| IBIS file stm32u595_599_5a5_5a9_tfbga169.ibs
[IBIS ver] 4.2
[File name] stm32u595_599_5a5_5a9_tfbga169.ibs
[File Rev] rev2.0
[Date]  11-09-2023
[Source] Data Created at STMicroelectronics
[Notes]  File originated from ELDO simulations.
[Disclaimer]  This information is for modeling purpose only and is
   not guaranteed. The information is subject to change without
   notice.
[Copyright] Copyright 2023 STMicroelectronics Inc.
|   Component stm32u595_599_5a5_5a9_tfbga169
[Component] stm32u595_599_5a5_5a9_tfbga169
[Manufacturer] STMicroelectronics
[Package]
| variable   typ   min   max
R_pkg  0  NA  NA
L_pkg  0  NA  NA
C_pkg  0  NA  NA
[Pin]   signal_name   model_name
A1  PE2  io8_100m_hslv_ft
A2  PI6  io8_spi_ft
A3  VDD  power
A4  VCAP  nc
A5  PG15  io8_100m_hslv_ft
A6  VDDIO2  power
A7  PG9  io8_100m_hslv_ft
A8  VDD  power
A9  PC11  io8_100m_hslv_ft
A10  PA15  nc
A11  VDD  power
A12  PI1  io8_spi_ft
A13  PH15  io8_spi_ft
B1  VDD  power
B2  VSS  gnd
B3  PI5  io8_100m_hslv_ft
B4  VSS  gnd
B5  PB6  io8_100m_i2c_ft
B6  PB4  io8_100m_i2c_ft
B7  PD6  io8_166m_hslv_ft
B8  VSS  gnd
B9  PD0  io8_100m_hslv_ft
B10  PI4  io8_spi_ft
B11  VSS  gnd
B12  PI0  io8_spi_ft
B13  PH12  io8_spi_ft
C1  VBAT  power
C2  PE4  io8_100m_hslv_tamp_ft
C3  PI7  io8_spi_ft
C4  PE1  io8_100m_hslv_ft
C5  PH3-BOOT0  nc
C6  PB5  io8_166m_hslv_ft
C7  PG10  io8_100m_hslv_ft
C8  PD4  io8_100m_hslv_ft
C9  PC10  io8_100m_ft
C10  PA14  io8_100m_ft
C11  PH14  io8_spi_ft
C12  PH13  io8_spi_ft
C13  PH10  io8_spi_ft
D1  PC14-OSC32_IN   nc
D2  PE5  io8_100m_hslv_tamp_ft
D3  PE3  io8_100m_hslv_tamp_ft
D4  PE0  io8_100m_hslv_ft
D5  PB9  io8_100m_i2c_ft
D6  PB3  io8_100m_i2c_ft
D7  PD7  io8_100m_hslv_ft
D8  PD3  io8_166m_hslv_ft
D9  PH11  io8_spi_ft
D10  PI3  io8_spi_ft
D11  PI2  io8_spi_ft
D12  PH8  io8_100m_hslv_ft
D13  VDD  power
E1  PC15-OSC32_OUT   nc
E2  PF0  io8_100m_hslv_ft
E3  PC13  io8_100m_ft
E4  PE6  io8_100m_hslv_tamp_ft
E5  PB8  io8_100m_i2c_ft
E6  PG12  io8_100m_hslv_ft
E7  PD5  io8_100m_hslv_ft
E8  PC12  io8_166m_hslv_ft
E9  PH9  io8_spi_ft
E10  PH4  io8_100m_hslv_ft
E11  PH6  io8_166m_hslv_ft
E12  VSS  gnd
E13  VDDUSB  power
F1  PF8  io8_100m_hslv_ft
F2  VSS  gnd
F3  PF1  io8_100m_hslv_ft
F4  PF2  io8_100m_hslv_ft
F5  PB7  io8_spi_hslv_ft
F6  PD1  io8_100m_hslv_ft
F7  PD2  io8_100m_ft
F8  PH7  io8_spi_hslv_ft
F9  PH5  io8_100m_i2c_ft
F10  PH2  io8_100m_hslv_ft
F11  PA10  io8_100m_usb_id
F12  PA13  io8_100m_ft
F13  PA12  io8_100m_ft
G1  VDD  power
G2  PF7  io8_100m_hslv_ft
G3  PF9  io8_100m_hslv_ft
G4  PF5  io8_spi_ft
G5  PF3  io8_100m_hslv_ft
G6  PF4  io8_spi_ft
G7  PA8  io8_166m_hslv_ft
G8  PG7  io8_100m_hslv_ft
G9  PC9  io8_100m_ft
G10  PC8  io8_100m_ft
G11  PA9  io8_100m_usb_vbus_ft
G12  PC7  io8_100m_ft
G13  PA11  io8_100m_ft
H1  PH0-OSC_IN  nc
H2  VSS  gnd
H3  NRST  nc
H4  PF10  io8_166m_hslv_ft
H5  OPAMP2_VINM  nc
H6  PF6  io8_100m_hslv_ft
H7  PG1  io8_100m_hslv_ft
H8  PE10  io8_166m_hslv_ft
H9  PG8  io8_100m_i2c_ft
H10  PG6  io8_100m_hslv_ft
H11  PG4  io8_100m_hslv_ft
H12  VDDIO2  power
H13  PC6  io8_100m_ft
J1  PH1-OSC_OUT   nc
J2  PC0  io8_100m_hslv_ft
J3  PC1  io8_spi_hslv_ft
J4  PC2  io8_100m_hslv_ft
J5  PA7  io8_100m_hslv_ft
J6  PG0  io8_100m_hslv_ft
J7  PE9  io8_166m_hslv_ft
J8  PG3  io8_100m_hslv_ft
J9  PG5  io8_100m_hslv_ft
J10  PD14  io8_100m_hslv_ft
J11  PD15  io8_100m_hslv_ft
J12  VSS  gnd
J13  VDD  power
K1  PC3  io8_100m_hslv_ft
K2  VSSA  nc
K3  PA0  io8_100m_hslv_tamp_ft
K4  PA5  io8_100m_ft
K5  PB0  io8_100m_hslv_ft
K6  PF12  io8_100m_hslv_ft
K7  PE8  io8_100m_hslv_ft
K8  PE14  io8_100m_hslv_ft
K9  PB10  io8_spi_hslv_ft
K10  PD12  io8_100m_hslv_ft
K11  PD10  io8_100m_hslv_ft
K12  PD13  io8_100m_hslv_ft
K13  PG2  io8_100m_hslv_ft
L1  VREFP  nc
L2  VDDA  nc
L3  PA1  io8_100m_hslv_tamp_ft
L4  PC4  io8_100m_hslv_ft
L5  PB2  io8_100m_hslv_tamp_ft
L6  PF14  io8_100m_hslv_ft
L7  PE7  io8_100m_hslv_ft
L8  PE13  io8_100m_hslv_ft
L9  PB11  io8_100m_hslv_ft
L10  PB12  io8_166m_hslv_ft
L11  PB15  nc
L12  PD8  io8_100m_hslv_ft
L13  PD9  io8_100m_hslv_ft
M1  OPAMP1_VINM  nc
M2  PA2  io8_100m_hslv_ft
M3  VSS  gnd
M4  PC5  io8_100m_tamp_ft
M5  PF11  io8_166m_hslv_ft
M6  PF13  io8_100m_hslv_ft
M7  VSS  gnd
M8  PE11  io8_100m_hslv_ft
M9  PE15  io8_100m_hslv_ft
M10  PG11  io8_100m_hslv_ft
M11  VSS  gnd
M12  PB14  io8_100m_i2c_ft
M13  PD11  io8_100m_hslv_ft
N1  PA4  io8_100m_hslv_ft
N2  PA3  io8_166m_hslv_ft
N3  VDD  power
N4  PA6  io8_100m_hslv_ft
N5  PB1  io8_100m_hslv_ft
N6  PF15  io8_100m_hslv_ft
N7  VDD  power
N8  PE12  io8_100m_hslv_ft
N9  PG14  io8_100m_hslv_ft
N10  PG13  io8_100m_hslv_ft
N11  VCAP  nc
N12  VDD  power
N13  PB13  io8_100m_i2c_ft
[Package Model]   481-tfbga-7x7-ldo-169-220908
[Pin Mapping]   pulldown_ref   pullup_ref   | Comment
A1  gndio  vddiom
A2  gndio  vddiom
A3  nc  vddiom
A4  nc  nc
A5  gndio  vddiom  | Depending on IO usage
| A5  gndio  vddio2  | Depending on IO usage
A6  nc  vddio2
A7  gndio  vddiom  | Depending on IO usage
| A7  gndio  vddio2  | Depending on IO usage
A8  nc  vddiom
A9  gndio  vddiom
A10  nc  nc
A11  nc  vddiom
A12  gndio  vddiom
A13  gndio  vddiom
B1  nc  vddiom
B2  gndio  nc
B3  gndio  vddiom
B4  gndio  nc
B5  gndio  vddiom
B6  gndio  vddiom
B7  gndio  vddiom
B8  gndio  nc
B9  gndio  vddiom
B10  gndio  vddiom
B11  gndio  nc
B12  gndio  vddiom
B13  gndio  vddiom
C1  nc  vsw
C2  gndio  vddiom
C3  gndio  vddiom
C4  gndio  vddiom
C5  nc  nc
C6  gndio  vddiom
C7  gndio  vddiom  | Depending on IO usage
| C7  gndio  vddio2  | Depending on IO usage
C8  gndio  vddiom
C9  gndio  vddiom
C10  gndio  vddiom
C11  gndio  vddiom
C12  gndio  vddiom
C13  gndio  vddiom
D1  nc  nc
D2  gndio  vddiom
D3  gndio  vddiom
D4  gndio  vddiom
D5  gndio  vddiom
D6  gndio  vddiom
D7  gndio  vddiom
D8  gndio  vddiom
D9  gndio  vddiom
D10  gndio  vddiom
D11  gndio  vddiom
D12  gndio  vddiom
D13  nc  vddiom
E1  nc  nc
E2  gndio  vddiom
E3  gndio  vddiom  | Depending on IO usage
| E3  gndio  vsw  | Depending on IO usage
E4  gndio  vddiom
E5  gndio  vddiom
E6  gndio  vddiom  | Depending on IO usage
| E6  gndio  vddio2  | Depending on IO usage
E7  gndio  vddiom
E8  gndio  vddiom
E9  gndio  vddiom
E10  gndio  vddiom
E11  gndio  vddiom
E12  gndio  nc
E13  nc  vddusb
F1  gndio  vddiom
F2  gndio  nc
F3  gndio  vddiom
F4  gndio  vddiom
F5  gndio  vddiom
F6  gndio  vddiom
F7  gndio  vddiom
F8  gndio  vddiom
F9  gndio  vddiom
F10  gndio  vddiom
F11  gndio  vddiom  | Depending on IO usage
| F11  gndio  vddusb  | Depending on IO usage
F12  gndio  vddiom  | Depending on IO usage
| F12  gndio  vddusb  | Depending on IO usage
F13  gndio  vddiom  | Depending on IO usage
| F13  gndio  vddusb  | Depending on IO usage
G1  nc  vddiom
G2  gndio  vddiom
G3  gndio  vddiom
G4  gndio  vddiom
G5  gndio  vddiom
G6  gndio  vddiom
G7  gndio  vddiom
G8  gndio  vddiom  | Depending on IO usage
| G8  gndio  vddio2  | Depending on IO usage
G9  gndio  vddiom
G10  gndio  vddiom
G11  gndio  vddiom  | Depending on IO usage
| G11  gndio  vddusb  | Depending on IO usage
G12  gndio  vddiom
G13  gndio  vddiom  | Depending on IO usage
| G13  gndio  vddusb  | Depending on IO usage
H1  nc  nc
H2  gndio  nc
H3  nc  nc
H4  gndio  vddiom
H5  nc  nc
H6  gndio  vddiom
H7  gndio  vddiom
H8  gndio  vddiom
H9  gndio  vddiom  | Depending on IO usage
| H9  gndio  vddio2  | Depending on IO usage
H10  gndio  vddiom  | Depending on IO usage
| H10  gndio  vddio2  | Depending on IO usage
H11  gndio  vddiom  | Depending on IO usage
| H11  gndio  vddio2  | Depending on IO usage
H12  nc  vddio2
H13  gndio  vddiom
J1  nc  nc
J2  gndio  vddiom
J3  gndio  vddiom
J4  gndio  vddiom
J5  gndio  vddiom
J6  gndio  vddiom
J7  gndio  vddiom
J8  gndio  vddiom  | Depending on IO usage
| J8  gndio  vddio2  | Depending on IO usage
J9  gndio  vddiom  | Depending on IO usage
| J9  gndio  vddio2  | Depending on IO usage
J10  gndio  vddiom
J11  gndio  vddiom
J12  gndio  nc
J13  nc  vddiom
K1  gndio  vddiom
K2  nc  nc
K3  gndio  vddiom
K4  gndio  vddiom
K5  gndio  vddiom
K6  gndio  vddiom
K7  gndio  vddiom
K8  gndio  vddiom
K9  gndio  vddiom
K10  gndio  vddiom
K11  gndio  vddiom
K12  gndio  vddiom
K13  gndio  vddiom  | Depending on IO usage
| K13  gndio  vddio2  | Depending on IO usage
L1  nc  nc
L2  nc  nc
L3  gndio  vddiom
L4  gndio  vddiom
L5  gndio  vddiom
L6  gndio  vddiom
L7  gndio  vddiom
L8  gndio  vddiom
L9  gndio  vddiom
L10  gndio  vddiom
L11  nc  nc
L12  gndio  vddiom
L13  gndio  vddiom
M1  nc  nc
M2  gndio  vddiom
M3  gndio  nc
M4  gndio  vddiom
M5  gndio  vddiom
M6  gndio  vddiom
M7  gndio  nc
M8  gndio  vddiom
M9  gndio  vddiom
M10  gndio  vddiom  | Depending on IO usage
| M10  gndio  vddio2  | Depending on IO usage
M11  gndio  nc
M12  gndio  vddiom
M13  gndio  vddiom
N1  gndio  vddiom
N2  gndio  vddiom
N3  nc  vddiom
N4  gndio  vddiom
N5  gndio  vddiom
N6  gndio  vddiom
N7  nc  vddiom
N8  gndio  vddiom
N9  gndio  vddiom  | Depending on IO usage
| N9  gndio  vddio2  | Depending on IO usage
N10  gndio  vddiom  | Depending on IO usage
| N10  gndio  vddio2  | Depending on IO usage
N11  nc  nc
N12  nc  vddiom
N13  gndio  vddiom
[Model Selector] io8_100m_ft
io8_100m_ft_hs_1v2  "IO8_FT 100MHz high speed @ 1.2V"
io8_100m_ft_fs_1v2  "IO8_FT 100MHz fast speed @ 1.2V"
io8_100m_ft_fs_pd_1v2  "IO8_FT 100MHz fast speed @ 1.2V pulldown"
io8_100m_ft_ms_1v2  "IO8_FT 100MHz med speed @ 1.2V"
io8_100m_ft_ms_pd_1v2  "IO8_FT 100MHz med speed @ 1.2V pulldown"
io8_100m_ft_ls_1v2  "IO8_FT 100MHz low speed @ 1.2V"
io8_100m_ft_ls_pd_1v2  "IO8_FT 100MHz low speed @ 1.2V pulldown"
io8_100m_ft_hs_1v8  "IO8_FT 100MHz high speed @ 1.8V"
io8_100m_ft_hs_pd_1v8  "IO8_FT 100MHz high speed @ 1.8V pulldown"
io8_100m_ft_fs_1v8  "IO8_FT 100MHz fast speed @ 1.8V"
io8_100m_ft_fs_pd_1v8  "IO8_FT 100MHz fast speed @ 1.8V pulldown"
io8_100m_ft_ms_1v8  "IO8_FT 100MHz med speed @ 1.8V"
io8_100m_ft_ms_pd_1v8  "IO8_FT 100MHz med speed @ 1.8V pulldown"
io8_100m_ft_ls_1v8  "IO8_FT 100MHz low speed @ 1.8V"
io8_100m_ft_ls_pd_1v8  "IO8_FT 100MHz low speed @ 1.8V pulldown"
io8_100m_ft_hs_3v3  "IO8_FT 100MHz high speed @ 3.3V"
io8_100m_ft_hs_pd_3v3  "IO8_FT 100MHz high speed @ 3.3V pulldown"
io8_100m_ft_fs_3v3  "IO8_FT 100MHz fast speed @ 3.3V"
io8_100m_ft_fs_pd_3v3  "IO8_FT 100MHz fast speed @ 3.3V pulldown"
io8_100m_ft_ms_3v3  "IO8_FT 100MHz med speed @ 3.3V"
io8_100m_ft_ms_pd_3v3  "IO8_FT 100MHz med speed @ 3.3V pulldown"
io8_100m_ft_ls_3v3  "IO8_FT 100MHz low speed @ 3.3V"
io8_100m_ft_ls_pd_3v3  "IO8_FT 100MHz low speed @ 3.3V pulldown"
[Model Selector] io8_100m_hslv_ft
io8_100m_ft_hs_1v2  "IO8_FT 100MHz high speed @ 1.2V"
io8_100m_ft_hs_pu_1v2  "IO8_FT 100MHz high speed @ 1.2V pullup"
io8_100m_ft_hs_pd_1v2  "IO8_FT 100MHz high speed @ 1.2V pulldown"
io8_100m_ft_fs_1v2  "IO8_FT 100MHz fast speed @ 1.2V"
io8_100m_ft_fs_pu_1v2  "IO8_FT 100MHz fast speed @ 1.2V pullup"
io8_100m_ft_fs_pd_1v2  "IO8_FT 100MHz fast speed @ 1.2V pulldown"
io8_100m_ft_ms_1v2  "IO8_FT 100MHz med speed @ 1.2V"
io8_100m_ft_ms_pu_1v2  "IO8_FT 100MHz med speed @ 1.2V pullup"
io8_100m_ft_ms_pd_1v2  "IO8_FT 100MHz med speed @ 1.2V pulldown"
io8_100m_ft_ls_1v2  "IO8_FT 100MHz low speed @ 1.2V"
io8_100m_ft_ls_pu_1v2  "IO8_FT 100MHz low speed @ 1.2V pullup"
io8_100m_ft_ls_pd_1v2  "IO8_FT 100MHz low speed @ 1.2V pulldown"
io8_100m_ft_hs_1v8  "IO8_FT 100MHz high speed @ 1.8V"
io8_100m_ft_hs_pu_1v8  "IO8_FT 100MHz high speed @ 1.8V pullup"
io8_100m_ft_hs_pd_1v8  "IO8_FT 100MHz high speed @ 1.8V pulldown"
io8_100m_ft_fs_1v8  "IO8_FT 100MHz fast speed @ 1.8V"
io8_100m_ft_fs_pu_1v8  "IO8_FT 100MHz fast speed @ 1.8V pullup"
io8_100m_ft_fs_pd_1v8  "IO8_FT 100MHz fast speed @ 1.8V pulldown"
io8_100m_ft_ms_1v8  "IO8_FT 100MHz med speed @ 1.8V"
io8_100m_ft_ms_pu_1v8  "IO8_FT 100MHz med speed @ 1.8V pullup"
io8_100m_ft_ms_pd_1v8  "IO8_FT 100MHz med speed @ 1.8V pulldown"
io8_100m_ft_ls_1v8  "IO8_FT 100MHz low speed @ 1.8V"
io8_100m_ft_ls_pu_1v8  "IO8_FT 100MHz low speed @ 1.8V pullup"
io8_100m_ft_ls_pd_1v8  "IO8_FT 100MHz low speed @ 1.8V pulldown"
io8_100m_ft_hs_3v3  "IO8_FT 100MHz high speed @ 3.3V"
io8_100m_ft_hs_pu_3v3  "IO8_FT 100MHz high speed @ 3.3V pullup"
io8_100m_ft_hs_pd_3v3  "IO8_FT 100MHz high speed @ 3.3V pulldown"
io8_100m_ft_fs_3v3  "IO8_FT 100MHz fast speed @ 3.3V"
io8_100m_ft_fs_pu_3v3  "IO8_FT 100MHz fast speed @ 3.3V pullup"
io8_100m_ft_fs_pd_3v3  "IO8_FT 100MHz fast speed @ 3.3V pulldown"
io8_100m_ft_ms_3v3  "IO8_FT 100MHz med speed @ 3.3V"
io8_100m_ft_ms_pu_3v3  "IO8_FT 100MHz med speed @ 3.3V pullup"
io8_100m_ft_ms_pd_3v3  "IO8_FT 100MHz med speed @ 3.3V pulldown"
io8_100m_ft_ls_3v3  "IO8_FT 100MHz low speed @ 3.3V"
io8_100m_ft_ls_pu_3v3  "IO8_FT 100MHz low speed @ 3.3V pullup"
io8_100m_ft_ls_pd_3v3  "IO8_FT 100MHz low speed @ 3.3V pulldown"
io8_100m_hslv_ft_hs_1v2  "IO8_FT 100MHz HSLV high speed @ 1.2V"
io8_100m_hslv_ft_hs_pu_1v2  "IO8_FT 100MHz HSLV high speed @ 1.2V pullup"
io8_100m_hslv_ft_hs_pd_1v2  "IO8_FT 100MHz HSLV high speed @ 1.2V pulldown"
io8_100m_hslv_ft_fs_1v2  "IO8_FT 100MHz HSLV fast speed @ 1.2V"
io8_100m_hslv_ft_fs_pu_1v2  "IO8_FT 100MHz HSLV fast speed @ 1.2V pullup"
io8_100m_hslv_ft_fs_pd_1v2  "IO8_FT 100MHz HSLV fast speed @ 1.2V pulldown"
io8_100m_hslv_ft_ms_1v2  "IO8_FT 100MHz HSLV med speed @ 1.2V"
io8_100m_hslv_ft_ms_pu_1v2  "IO8_FT 100MHz HSLV med speed @ 1.2V pullup"
io8_100m_hslv_ft_ms_pd_1v2  "IO8_FT 100MHz HSLV med speed @ 1.2V pulldown"
io8_100m_hslv_ft_ls_1v2  "IO8_FT 100MHz HSLV low speed @ 1.2V"
io8_100m_hslv_ft_ls_pu_1v2  "IO8_FT 100MHz HSLV low speed @ 1.2V pullup"
io8_100m_hslv_ft_ls_pd_1v2  "IO8_FT 100MHz HSLV low speed @ 1.2V pulldown"
io8_100m_hslv_ft_hs_1v8  "IO8_FT 100MHz HSLV high speed @ 1.8V"
io8_100m_hslv_ft_hs_pu_1v8  "IO8_FT 100MHz HSLV high speed @ 1.8V pullup"
io8_100m_hslv_ft_hs_pd_1v8  "IO8_FT 100MHz HSLV high speed @ 1.8V pulldown"
io8_100m_hslv_ft_fs_1v8  "IO8_FT 100MHz HSLV fast speed @ 1.8V"
io8_100m_hslv_ft_fs_pu_1v8  "IO8_FT 100MHz HSLV fast speed @ 1.8V pullup"
io8_100m_hslv_ft_fs_pd_1v8  "IO8_FT 100MHz HSLV fast speed @ 1.8V pulldown"
io8_100m_hslv_ft_ms_1v8  "IO8_FT 100MHz HSLV med speed @ 1.8V"
io8_100m_hslv_ft_ms_pu_1v8  "IO8_FT 100MHz HSLV med speed @ 1.8V pullup"
io8_100m_hslv_ft_ms_pd_1v8  "IO8_FT 100MHz HSLV med speed @ 1.8V pulldown"
io8_100m_hslv_ft_ls_1v8  "IO8_FT 100MHz HSLV low speed @ 1.8V"
io8_100m_hslv_ft_ls_pu_1v8  "IO8_FT 100MHz HSLV low speed @ 1.8V pullup"
io8_100m_hslv_ft_ls_pd_1v8  "IO8_FT 100MHz HSLV low speed @ 1.8V pulldown"
io8_100m_hslv_ft_hs_2v5  "IO8_FT 100MHz HSLV high speed @ 2.5V"
io8_100m_hslv_ft_hs_pu_2v5  "IO8_FT 100MHz HSLV high speed @ 2.5V pullup"
io8_100m_hslv_ft_hs_pd_2v5  "IO8_FT 100MHz HSLV high speed @ 2.5V pulldown"
io8_100m_hslv_ft_fs_2v5  "IO8_FT 100MHz HSLV fast speed @ 2.5V"
io8_100m_hslv_ft_fs_pu_2v5  "IO8_FT 100MHz HSLV fast speed @ 2.5V pullup"
io8_100m_hslv_ft_fs_pd_2v5  "IO8_FT 100MHz HSLV fast speed @ 2.5V pulldown"
io8_100m_hslv_ft_ms_2v5  "IO8_FT 100MHz HSLV med speed @ 2.5V"
io8_100m_hslv_ft_ms_pu_2v5  "IO8_FT 100MHz HSLV med speed @ 2.5V pullup"
io8_100m_hslv_ft_ms_pd_2v5  "IO8_FT 100MHz HSLV med speed @ 2.5V pulldown"
io8_100m_hslv_ft_ls_2v5  "IO8_FT 100MHz HSLV low speed @ 2.5V"
io8_100m_hslv_ft_ls_pu_2v5  "IO8_FT 100MHz HSLV low speed @ 2.5V pullup"
io8_100m_hslv_ft_ls_pd_2v5  "IO8_FT 100MHz HSLV low speed @ 2.5V pulldown"
[Model Selector] io8_100m_hslv_tamp_ft
io8_100m_ft_hs_1v2  "IO8_FT 100MHz high speed @ 1.2V"
io8_100m_ft_hs_pu_1v2  "IO8_FT 100MHz high speed @ 1.2V pullup"
io8_100m_ft_hs_pd_1v2  "IO8_FT 100MHz high speed @ 1.2V pulldown"
io8_100m_ft_fs_1v2  "IO8_FT 100MHz fast speed @ 1.2V"
io8_100m_ft_fs_pu_1v2  "IO8_FT 100MHz fast speed @ 1.2V pullup"
io8_100m_ft_fs_pd_1v2  "IO8_FT 100MHz fast speed @ 1.2V pulldown"
io8_100m_ft_ms_1v2  "IO8_FT 100MHz med speed @ 1.2V"
io8_100m_ft_ms_pu_1v2  "IO8_FT 100MHz med speed @ 1.2V pullup"
io8_100m_ft_ms_pd_1v2  "IO8_FT 100MHz med speed @ 1.2V pulldown"
io8_100m_ft_ls_1v2  "IO8_FT 100MHz low speed @ 1.2V"
io8_100m_ft_ls_pu_1v2  "IO8_FT 100MHz low speed @ 1.2V pullup"
io8_100m_ft_ls_pd_1v2  "IO8_FT 100MHz low speed @ 1.2V pulldown"
io8_100m_ft_hs_1v8  "IO8_FT 100MHz high speed @ 1.8V"
io8_100m_ft_hs_pu_1v8  "IO8_FT 100MHz high speed @ 1.8V pullup"
io8_100m_ft_hs_pd_1v8  "IO8_FT 100MHz high speed @ 1.8V pulldown"
io8_100m_ft_fs_1v8  "IO8_FT 100MHz fast speed @ 1.8V"
io8_100m_ft_fs_pu_1v8  "IO8_FT 100MHz fast speed @ 1.8V pullup"
io8_100m_ft_fs_pd_1v8  "IO8_FT 100MHz fast speed @ 1.8V pulldown"
io8_100m_ft_ms_1v8  "IO8_FT 100MHz med speed @ 1.8V"
io8_100m_ft_ms_pu_1v8  "IO8_FT 100MHz med speed @ 1.8V pullup"
io8_100m_ft_ms_pd_1v8  "IO8_FT 100MHz med speed @ 1.8V pulldown"
io8_100m_ft_ls_1v8  "IO8_FT 100MHz low speed @ 1.8V"
io8_100m_ft_ls_pu_1v8  "IO8_FT 100MHz low speed @ 1.8V pullup"
io8_100m_ft_ls_pd_1v8  "IO8_FT 100MHz low speed @ 1.8V pulldown"
io8_100m_ft_hs_3v3  "IO8_FT 100MHz high speed @ 3.3V"
io8_100m_ft_hs_pu_3v3  "IO8_FT 100MHz high speed @ 3.3V pullup"
io8_100m_ft_hs_pd_3v3  "IO8_FT 100MHz high speed @ 3.3V pulldown"
io8_100m_ft_fs_3v3  "IO8_FT 100MHz fast speed @ 3.3V"
io8_100m_ft_fs_pu_3v3  "IO8_FT 100MHz fast speed @ 3.3V pullup"
io8_100m_ft_fs_pd_3v3  "IO8_FT 100MHz fast speed @ 3.3V pulldown"
io8_100m_ft_ms_3v3  "IO8_FT 100MHz med speed @ 3.3V"
io8_100m_ft_ms_pu_3v3  "IO8_FT 100MHz med speed @ 3.3V pullup"
io8_100m_ft_ms_pd_3v3  "IO8_FT 100MHz med speed @ 3.3V pulldown"
io8_100m_ft_ls_3v3  "IO8_FT 100MHz low speed @ 3.3V"
io8_100m_ft_ls_pu_3v3  "IO8_FT 100MHz low speed @ 3.3V pullup"
io8_100m_ft_ls_pd_3v3  "IO8_FT 100MHz low speed @ 3.3V pulldown"
io8_100m_hslv_ft_hs_1v2  "IO8_FT 100MHz HSLV high speed @ 1.2V"
io8_100m_hslv_ft_hs_pu_1v2  "IO8_FT 100MHz HSLV high speed @ 1.2V pullup"
io8_100m_hslv_ft_hs_pd_1v2  "IO8_FT 100MHz HSLV high speed @ 1.2V pulldown"
io8_100m_hslv_ft_fs_1v2  "IO8_FT 100MHz HSLV fast speed @ 1.2V"
io8_100m_hslv_ft_fs_pu_1v2  "IO8_FT 100MHz HSLV fast speed @ 1.2V pullup"
io8_100m_hslv_ft_fs_pd_1v2  "IO8_FT 100MHz HSLV fast speed @ 1.2V pulldown"
io8_100m_hslv_ft_ms_1v2  "IO8_FT 100MHz HSLV med speed @ 1.2V"
io8_100m_hslv_ft_ms_pu_1v2  "IO8_FT 100MHz HSLV med speed @ 1.2V pullup"
io8_100m_hslv_ft_ms_pd_1v2  "IO8_FT 100MHz HSLV med speed @ 1.2V pulldown"
io8_100m_hslv_ft_ls_1v2  "IO8_FT 100MHz HSLV low speed @ 1.2V"
io8_100m_hslv_ft_ls_pu_1v2  "IO8_FT 100MHz HSLV low speed @ 1.2V pullup"
io8_100m_hslv_ft_ls_pd_1v2  "IO8_FT 100MHz HSLV low speed @ 1.2V pulldown"
io8_100m_hslv_ft_hs_1v8  "IO8_FT 100MHz HSLV high speed @ 1.8V"
io8_100m_hslv_ft_hs_pu_1v8  "IO8_FT 100MHz HSLV high speed @ 1.8V pullup"
io8_100m_hslv_ft_hs_pd_1v8  "IO8_FT 100MHz HSLV high speed @ 1.8V pulldown"
io8_100m_hslv_ft_fs_1v8  "IO8_FT 100MHz HSLV fast speed @ 1.8V"
io8_100m_hslv_ft_fs_pu_1v8  "IO8_FT 100MHz HSLV fast speed @ 1.8V pullup"
io8_100m_hslv_ft_fs_pd_1v8  "IO8_FT 100MHz HSLV fast speed @ 1.8V pulldown"
io8_100m_hslv_ft_ms_1v8  "IO8_FT 100MHz HSLV med speed @ 1.8V"
io8_100m_hslv_ft_ms_pu_1v8  "IO8_FT 100MHz HSLV med speed @ 1.8V pullup"
io8_100m_hslv_ft_ms_pd_1v8  "IO8_FT 100MHz HSLV med speed @ 1.8V pulldown"
io8_100m_hslv_ft_ls_1v8  "IO8_FT 100MHz HSLV low speed @ 1.8V"
io8_100m_hslv_ft_ls_pu_1v8  "IO8_FT 100MHz HSLV low speed @ 1.8V pullup"
io8_100m_hslv_ft_ls_pd_1v8  "IO8_FT 100MHz HSLV low speed @ 1.8V pulldown"
io8_100m_hslv_ft_hs_2v5  "IO8_FT 100MHz HSLV high speed @ 2.5V"
io8_100m_hslv_ft_hs_pu_2v5  "IO8_FT 100MHz HSLV high speed @ 2.5V pullup"
io8_100m_hslv_ft_hs_pd_2v5  "IO8_FT 100MHz HSLV high speed @ 2.5V pulldown"
io8_100m_hslv_ft_fs_2v5  "IO8_FT 100MHz HSLV fast speed @ 2.5V"
io8_100m_hslv_ft_fs_pu_2v5  "IO8_FT 100MHz HSLV fast speed @ 2.5V pullup"
io8_100m_hslv_ft_fs_pd_2v5  "IO8_FT 100MHz HSLV fast speed @ 2.5V pulldown"
io8_100m_hslv_ft_ms_2v5  "IO8_FT 100MHz HSLV med speed @ 2.5V"
io8_100m_hslv_ft_ms_pu_2v5  "IO8_FT 100MHz HSLV med speed @ 2.5V pullup"
io8_100m_hslv_ft_ms_pd_2v5  "IO8_FT 100MHz HSLV med speed @ 2.5V pulldown"
io8_100m_hslv_ft_ls_2v5  "IO8_FT 100MHz HSLV low speed @ 2.5V"
io8_100m_hslv_ft_ls_pu_2v5  "IO8_FT 100MHz HSLV low speed @ 2.5V pullup"
io8_100m_hslv_ft_ls_pd_2v5  "IO8_FT 100MHz HSLV low speed @ 2.5V pulldown"
io8_ft_v33_hs_1v2  "IO8_FT_V33 high speed @ 1.2V"
io8_ft_v33_hs_pu_1v2  "IO8_FT_V33 high speed @ 1.2V pullup"
io8_ft_v33_hs_pd_1v2  "IO8_FT_V33 high speed @ 1.2V pulldown"
io8_ft_v33_fs_1v2  "IO8_FT_V33 fast speed @ 1.2V"
io8_ft_v33_fs_pu_1v2  "IO8_FT_V33 fast speed @ 1.2V pullup"
io8_ft_v33_fs_pd_1v2  "IO8_FT_V33 fast speed @ 1.2V pulldown"
io8_ft_v33_ms_1v2  "IO8_FT_V33 med speed @ 1.2V"
io8_ft_v33_ms_pu_1v2  "IO8_FT_V33 med speed @ 1.2V pullup"
io8_ft_v33_ms_pd_1v2  "IO8_FT_V33 med speed @ 1.2V pulldown"
io8_ft_v33_ls_1v2  "IO8_FT_V33 low speed @ 1.2V"
io8_ft_v33_ls_pu_1v2  "IO8_FT_V33 low speed @ 1.2V pullup"
io8_ft_v33_ls_pd_1v2  "IO8_FT_V33 low speed @ 1.2V pulldown"
io8_ft_v33_hs_1v8  "IO8_FT_V33 high speed @ 1.8V"
io8_ft_v33_hs_pu_1v8  "IO8_FT_V33 high speed @ 1.8V pullup"
io8_ft_v33_hs_pd_1v8  "IO8_FT_V33 high speed @ 1.8V pulldown"
io8_ft_v33_fs_1v8  "IO8_FT_V33 fast speed @ 1.8V"
io8_ft_v33_fs_pu_1v8  "IO8_FT_V33 fast speed @ 1.8V pullup"
io8_ft_v33_fs_pd_1v8  "IO8_FT_V33 fast speed @ 1.8V pulldown"
io8_ft_v33_ms_1v8  "IO8_FT_V33 med speed @ 1.8V"
io8_ft_v33_ms_pu_1v8  "IO8_FT_V33 med speed @ 1.8V pullup"
io8_ft_v33_ms_pd_1v8  "IO8_FT_V33 med speed @ 1.8V pulldown"
io8_ft_v33_ls_1v8  "IO8_FT_V33 low speed @ 1.8V"
io8_ft_v33_ls_pu_1v8  "IO8_FT_V33 low speed @ 1.8V pullup"
io8_ft_v33_ls_pd_1v8  "IO8_FT_V33 low speed @ 1.8V pulldown"
io8_ft_v33_hs_3v3  "IO8_FT_V33 high speed @ 3.3V"
io8_ft_v33_hs_pu_3v3  "IO8_FT_V33 high speed @ 3.3V pullup"
io8_ft_v33_hs_pd_3v3  "IO8_FT_V33 high speed @ 3.3V pulldown"
io8_ft_v33_fs_3v3  "IO8_FT_V33 fast speed @ 3.3V"
io8_ft_v33_fs_pu_3v3  "IO8_FT_V33 fast speed @ 3.3V pullup"
io8_ft_v33_fs_pd_3v3  "IO8_FT_V33 fast speed @ 3.3V pulldown"
io8_ft_v33_ms_3v3  "IO8_FT_V33 med speed @ 3.3V"
io8_ft_v33_ms_pu_3v3  "IO8_FT_V33 med speed @ 3.3V pullup"
io8_ft_v33_ms_pd_3v3  "IO8_FT_V33 med speed @ 3.3V pulldown"
io8_ft_v33_ls_3v3  "IO8_FT_V33 low speed @ 3.3V"
io8_ft_v33_ls_pu_3v3  "IO8_FT_V33 low speed @ 3.3V pullup"
io8_ft_v33_ls_pd_3v3  "IO8_FT_V33 low speed @ 3.3V pulldown"
[Model Selector] io8_100m_i2c_ft
io8_100m_ft_hs_1v2  "IO8_FT 100MHz high speed @ 1.2V"
io8_100m_ft_hs_pu_1v2  "IO8_FT 100MHz high speed @ 1.2V pullup"
io8_100m_ft_hs_pd_1v2  "IO8_FT 100MHz high speed @ 1.2V pulldown"
io8_100m_ft_fs_1v2  "IO8_FT 100MHz fast speed @ 1.2V"
io8_100m_ft_fs_pu_1v2  "IO8_FT 100MHz fast speed @ 1.2V pullup"
io8_100m_ft_fs_pd_1v2  "IO8_FT 100MHz fast speed @ 1.2V pulldown"
io8_100m_ft_ms_1v2  "IO8_FT 100MHz med speed @ 1.2V"
io8_100m_ft_ms_pu_1v2  "IO8_FT 100MHz med speed @ 1.2V pullup"
io8_100m_ft_ms_pd_1v2  "IO8_FT 100MHz med speed @ 1.2V pulldown"
io8_100m_ft_ls_1v2  "IO8_FT 100MHz low speed @ 1.2V"
io8_100m_ft_ls_pu_1v2  "IO8_FT 100MHz low speed @ 1.2V pullup"
io8_100m_ft_ls_pd_1v2  "IO8_FT 100MHz low speed @ 1.2V pulldown"
io8_100m_ft_hs_1v8  "IO8_FT 100MHz high speed @ 1.8V"
io8_100m_ft_hs_pu_1v8  "IO8_FT 100MHz high speed @ 1.8V pullup"
io8_100m_ft_hs_pd_1v8  "IO8_FT 100MHz high speed @ 1.8V pulldown"
io8_100m_ft_fs_1v8  "IO8_FT 100MHz fast speed @ 1.8V"
io8_100m_ft_fs_pu_1v8  "IO8_FT 100MHz fast speed @ 1.8V pullup"
io8_100m_ft_fs_pd_1v8  "IO8_FT 100MHz fast speed @ 1.8V pulldown"
io8_100m_ft_ms_1v8  "IO8_FT 100MHz med speed @ 1.8V"
io8_100m_ft_ms_pu_1v8  "IO8_FT 100MHz med speed @ 1.8V pullup"
io8_100m_ft_ms_pd_1v8  "IO8_FT 100MHz med speed @ 1.8V pulldown"
io8_100m_ft_ls_1v8  "IO8_FT 100MHz low speed @ 1.8V"
io8_100m_ft_ls_pu_1v8  "IO8_FT 100MHz low speed @ 1.8V pullup"
io8_100m_ft_ls_pd_1v8  "IO8_FT 100MHz low speed @ 1.8V pulldown"
io8_100m_ft_hs_3v3  "IO8_FT 100MHz high speed @ 3.3V"
io8_100m_ft_hs_pu_3v3  "IO8_FT 100MHz high speed @ 3.3V pullup"
io8_100m_ft_hs_pd_3v3  "IO8_FT 100MHz high speed @ 3.3V pulldown"
io8_100m_ft_fs_3v3  "IO8_FT 100MHz fast speed @ 3.3V"
io8_100m_ft_fs_pu_3v3  "IO8_FT 100MHz fast speed @ 3.3V pullup"
io8_100m_ft_fs_pd_3v3  "IO8_FT 100MHz fast speed @ 3.3V pulldown"
io8_100m_ft_ms_3v3  "IO8_FT 100MHz med speed @ 3.3V"
io8_100m_ft_ms_pu_3v3  "IO8_FT 100MHz med speed @ 3.3V pullup"
io8_100m_ft_ms_pd_3v3  "IO8_FT 100MHz med speed @ 3.3V pulldown"
io8_100m_ft_ls_3v3  "IO8_FT 100MHz low speed @ 3.3V"
io8_100m_ft_ls_pu_3v3  "IO8_FT 100MHz low speed @ 3.3V pullup"
io8_100m_ft_ls_pd_3v3  "IO8_FT 100MHz low speed @ 3.3V pulldown"
io8_100m_i2c_ft_1v2  "IO8_FT 100MHz I2C @ 1.2V"
io8_100m_i2c_ft_pu_1v2  "IO8_FT 100MHz I2C @ 1.2V pullup"
io8_100m_i2c_ft_pd_1v2  "IO8_FT 100MHz I2C @ 1.2V pulldown"
io8_100m_i2c_ft_1v8  "IO8_FT 100MHz I2C @ 1.8V"
io8_100m_i2c_ft_pu_1v8  "IO8_FT 100MHz I2C @ 1.8V pullup"
io8_100m_i2c_ft_pd_1v8  "IO8_FT 100MHz I2C @ 1,8V pulldown"
io8_100m_i2c_ft_3v3  "IO8_FT 100MHz I2C @ 3.3V"
io8_100m_i2c_ft_pu_3v3  "IO8_FT 100MHz I2C HSLV @ 3.3V pullup"
io8_100m_i2c_ft_pd_3v3  "IO8_FT 100MHz I2C @ 3.3V pulldown"
[Model Selector] io8_100m_tamp_ft
io8_100m_ft_hs_1v2  "IO8_FT 100MHz high speed @ 1.2V"
io8_100m_ft_hs_pu_1v2  "IO8_FT 100MHz high speed @ 1.2V pullup"
io8_100m_ft_hs_pd_1v2  "IO8_FT 100MHz high speed @ 1.2V pulldown"
io8_100m_ft_fs_1v2  "IO8_FT 100MHz fast speed @ 1.2V"
io8_100m_ft_fs_pu_1v2  "IO8_FT 100MHz fast speed @ 1.2V pullup"
io8_100m_ft_fs_pd_1v2  "IO8_FT 100MHz fast speed @ 1.2V pulldown"
io8_100m_ft_ms_1v2  "IO8_FT 100MHz med speed @ 1.2V"
io8_100m_ft_ms_pu_1v2  "IO8_FT 100MHz med speed @ 1.2V pullup"
io8_100m_ft_ms_pd_1v2  "IO8_FT 100MHz med speed @ 1.2V pulldown"
io8_100m_ft_ls_1v2  "IO8_FT 100MHz low speed @ 1.2V"
io8_100m_ft_ls_pu_1v2  "IO8_FT 100MHz low speed @ 1.2V pullup"
io8_100m_ft_ls_pd_1v2  "IO8_FT 100MHz low speed @ 1.2V pulldown"
io8_100m_ft_hs_1v8  "IO8_FT 100MHz high speed @ 1.8V"
io8_100m_ft_hs_pu_1v8  "IO8_FT 100MHz high speed @ 1.8V pullup"
io8_100m_ft_hs_pd_1v8  "IO8_FT 100MHz high speed @ 1.8V pulldown"
io8_100m_ft_fs_1v8  "IO8_FT 100MHz fast speed @ 1.8V"
io8_100m_ft_fs_pu_1v8  "IO8_FT 100MHz fast speed @ 1.8V pullup"
io8_100m_ft_fs_pd_1v8  "IO8_FT 100MHz fast speed @ 1.8V pulldown"
io8_100m_ft_ms_1v8  "IO8_FT 100MHz med speed @ 1.8V"
io8_100m_ft_ms_pu_1v8  "IO8_FT 100MHz med speed @ 1.8V pullup"
io8_100m_ft_ms_pd_1v8  "IO8_FT 100MHz med speed @ 1.8V pulldown"
io8_100m_ft_ls_1v8  "IO8_FT 100MHz low speed @ 1.8V"
io8_100m_ft_ls_pu_1v8  "IO8_FT 100MHz low speed @ 1.8V pullup"
io8_100m_ft_ls_pd_1v8  "IO8_FT 100MHz low speed @ 1.8V pulldown"
io8_100m_ft_hs_3v3  "IO8_FT 100MHz high speed @ 3.3V"
io8_100m_ft_hs_pu_3v3  "IO8_FT 100MHz high speed @ 3.3V pullup"
io8_100m_ft_hs_pd_3v3  "IO8_FT 100MHz high speed @ 3.3V pulldown"
io8_100m_ft_fs_3v3  "IO8_FT 100MHz fast speed @ 3.3V"
io8_100m_ft_fs_pu_3v3  "IO8_FT 100MHz fast speed @ 3.3V pullup"
io8_100m_ft_fs_pd_3v3  "IO8_FT 100MHz fast speed @ 3.3V pulldown"
io8_100m_ft_ms_3v3  "IO8_FT 100MHz med speed @ 3.3V"
io8_100m_ft_ms_pu_3v3  "IO8_FT 100MHz med speed @ 3.3V pullup"
io8_100m_ft_ms_pd_3v3  "IO8_FT 100MHz med speed @ 3.3V pulldown"
io8_100m_ft_ls_3v3  "IO8_FT 100MHz low speed @ 3.3V"
io8_100m_ft_ls_pu_3v3  "IO8_FT 100MHz low speed @ 3.3V pullup"
io8_100m_ft_ls_pd_3v3  "IO8_FT 100MHz low speed @ 3.3V pulldown"
io8_ft_v33_hs_1v2  "IO8_FT_V33 high speed @ 1.2V"
io8_ft_v33_hs_pu_1v2  "IO8_FT_V33 high speed @ 1.2V pullup"
io8_ft_v33_hs_pd_1v2  "IO8_FT_V33 high speed @ 1.2V pulldown"
io8_ft_v33_fs_1v2  "IO8_FT_V33 fast speed @ 1.2V"
io8_ft_v33_fs_pu_1v2  "IO8_FT_V33 fast speed @ 1.2V pullup"
io8_ft_v33_fs_pd_1v2  "IO8_FT_V33 fast speed @ 1.2V pulldown"
io8_ft_v33_ms_1v2  "IO8_FT_V33 med speed @ 1.2V"
io8_ft_v33_ms_pu_1v2  "IO8_FT_V33 med speed @ 1.2V pullup"
io8_ft_v33_ms_pd_1v2  "IO8_FT_V33 med speed @ 1.2V pulldown"
io8_ft_v33_ls_1v2  "IO8_FT_V33 low speed @ 1.2V"
io8_ft_v33_ls_pu_1v2  "IO8_FT_V33 low speed @ 1.2V pullup"
io8_ft_v33_ls_pd_1v2  "IO8_FT_V33 low speed @ 1.2V pulldown"
io8_ft_v33_hs_1v8  "IO8_FT_V33 high speed @ 1.8V"
io8_ft_v33_hs_pu_1v8  "IO8_FT_V33 high speed @ 1.8V pullup"
io8_ft_v33_hs_pd_1v8  "IO8_FT_V33 high speed @ 1.8V pulldown"
io8_ft_v33_fs_1v8  "IO8_FT_V33 fast speed @ 1.8V"
io8_ft_v33_fs_pu_1v8  "IO8_FT_V33 fast speed @ 1.8V pullup"
io8_ft_v33_fs_pd_1v8  "IO8_FT_V33 fast speed @ 1.8V pulldown"
io8_ft_v33_ms_1v8  "IO8_FT_V33 med speed @ 1.8V"
io8_ft_v33_ms_pu_1v8  "IO8_FT_V33 med speed @ 1.8V pullup"
io8_ft_v33_ms_pd_1v8  "IO8_FT_V33 med speed @ 1.8V pulldown"
io8_ft_v33_ls_1v8  "IO8_FT_V33 low speed @ 1.8V"
io8_ft_v33_ls_pu_1v8  "IO8_FT_V33 low speed @ 1.8V pullup"
io8_ft_v33_ls_pd_1v8  "IO8_FT_V33 low speed @ 1.8V pulldown"
io8_ft_v33_hs_3v3  "IO8_FT_V33 high speed @ 3.3V"
io8_ft_v33_hs_pu_3v3  "IO8_FT_V33 high speed @ 3.3V pullup"
io8_ft_v33_hs_pd_3v3  "IO8_FT_V33 high speed @ 3.3V pulldown"
io8_ft_v33_fs_3v3  "IO8_FT_V33 fast speed @ 3.3V"
io8_ft_v33_fs_pu_3v3  "IO8_FT_V33 fast speed @ 3.3V pullup"
io8_ft_v33_fs_pd_3v3  "IO8_FT_V33 fast speed @ 3.3V pulldown"
io8_ft_v33_ms_3v3  "IO8_FT_V33 med speed @ 3.3V"
io8_ft_v33_ms_pu_3v3  "IO8_FT_V33 med speed @ 3.3V pullup"
io8_ft_v33_ms_pd_3v3  "IO8_FT_V33 med speed @ 3.3V pulldown"
io8_ft_v33_ls_3v3  "IO8_FT_V33 low speed @ 3.3V"
io8_ft_v33_ls_pu_3v3  "IO8_FT_V33 low speed @ 3.3V pullup"
io8_ft_v33_ls_pd_3v3  "IO8_FT_V33 low speed @ 3.3V pulldown"
[Model Selector] io8_100m_usb_id
io8_100m_ft_hs_1v2  "IO8_FT 100MHz high speed @ 1.2V"
io8_100m_ft_hs_pu_1v2  "IO8_FT 100MHz high speed @ 1.2V pullup"
io8_100m_ft_hs_pd_1v2  "IO8_FT 100MHz high speed @ 1.2V pulldown"
io8_100m_ft_fs_1v2  "IO8_FT 100MHz fast speed @ 1.2V"
io8_100m_ft_fs_pu_1v2  "IO8_FT 100MHz fast speed @ 1.2V pullup"
io8_100m_ft_fs_pd_1v2  "IO8_FT 100MHz fast speed @ 1.2V pulldown"
io8_100m_ft_ms_1v2  "IO8_FT 100MHz med speed @ 1.2V"
io8_100m_ft_ms_pu_1v2  "IO8_FT 100MHz med speed @ 1.2V pullup"
io8_100m_ft_ms_pd_1v2  "IO8_FT 100MHz med speed @ 1.2V pulldown"
io8_100m_ft_ls_1v2  "IO8_FT 100MHz low speed @ 1.2V"
io8_100m_ft_ls_pu_1v2  "IO8_FT 100MHz low speed @ 1.2V pullup"
io8_100m_ft_ls_pd_1v2  "IO8_FT 100MHz low speed @ 1.2V pulldown"
io8_100m_ft_hs_1v8  "IO8_FT 100MHz high speed @ 1.8V"
io8_100m_ft_hs_pu_1v8  "IO8_FT 100MHz high speed @ 1.8V pullup"
io8_100m_ft_hs_pd_1v8  "IO8_FT 100MHz high speed @ 1.8V pulldown"
io8_100m_ft_fs_1v8  "IO8_FT 100MHz fast speed @ 1.8V"
io8_100m_ft_fs_pu_1v8  "IO8_FT 100MHz fast speed @ 1.8V pullup"
io8_100m_ft_fs_pd_1v8  "IO8_FT 100MHz fast speed @ 1.8V pulldown"
io8_100m_ft_ms_1v8  "IO8_FT 100MHz med speed @ 1.8V"
io8_100m_ft_ms_pu_1v8  "IO8_FT 100MHz med speed @ 1.8V pullup"
io8_100m_ft_ms_pd_1v8  "IO8_FT 100MHz med speed @ 1.8V pulldown"
io8_100m_ft_ls_1v8  "IO8_FT 100MHz low speed @ 1.8V"
io8_100m_ft_ls_pu_1v8  "IO8_FT 100MHz low speed @ 1.8V pullup"
io8_100m_ft_ls_pd_1v8  "IO8_FT 100MHz low speed @ 1.8V pulldown"
io8_100m_ft_hs_3v3  "IO8_FT 100MHz high speed @ 3.3V"
io8_100m_ft_hs_pu_3v3  "IO8_FT 100MHz high speed @ 3.3V pullup"
io8_100m_ft_hs_pd_3v3  "IO8_FT 100MHz high speed @ 3.3V pulldown"
io8_100m_ft_fs_3v3  "IO8_FT 100MHz fast speed @ 3.3V"
io8_100m_ft_fs_pu_3v3  "IO8_FT 100MHz fast speed @ 3.3V pullup"
io8_100m_ft_fs_pd_3v3  "IO8_FT 100MHz fast speed @ 3.3V pulldown"
io8_100m_ft_ms_3v3  "IO8_FT 100MHz med speed @ 3.3V"
io8_100m_ft_ms_pu_3v3  "IO8_FT 100MHz med speed @ 3.3V pullup"
io8_100m_ft_ms_pd_3v3  "IO8_FT 100MHz med speed @ 3.3V pulldown"
io8_100m_ft_ls_3v3  "IO8_FT 100MHz low speed @ 3.3V"
io8_100m_ft_ls_pu_3v3  "IO8_FT 100MHz low speed @ 3.3V pullup"
io8_100m_ft_ls_pd_3v3  "IO8_FT 100MHz low speed @ 3.3V pulldown"
io8usb_id_nopu  "IOUSB ID @ 3.3V"
io8usb_id_pu  "IOUSB ID @ 3.3V pullup"
[Model Selector] io8_100m_usb_vbus_ft
io8_100m_ft_hs_1v2  "IO8_FT 100MHz high speed @ 1.2V"
io8_100m_ft_hs_pu_1v2  "IO8_FT 100MHz high speed @ 1.2V pullup"
io8_100m_ft_hs_pd_1v2  "IO8_FT 100MHz high speed @ 1.2V pulldown"
io8_100m_ft_fs_1v2  "IO8_FT 100MHz fast speed @ 1.2V"
io8_100m_ft_fs_pu_1v2  "IO8_FT 100MHz fast speed @ 1.2V pullup"
io8_100m_ft_fs_pd_1v2  "IO8_FT 100MHz fast speed @ 1.2V pulldown"
io8_100m_ft_ms_1v2  "IO8_FT 100MHz med speed @ 1.2V"
io8_100m_ft_ms_pu_1v2  "IO8_FT 100MHz med speed @ 1.2V pullup"
io8_100m_ft_ms_pd_1v2  "IO8_FT 100MHz med speed @ 1.2V pulldown"
io8_100m_ft_ls_1v2  "IO8_FT 100MHz low speed @ 1.2V"
io8_100m_ft_ls_pu_1v2  "IO8_FT 100MHz low speed @ 1.2V pullup"
io8_100m_ft_ls_pd_1v2  "IO8_FT 100MHz low speed @ 1.2V pulldown"
io8_100m_ft_hs_1v8  "IO8_FT 100MHz high speed @ 1.8V"
io8_100m_ft_hs_pu_1v8  "IO8_FT 100MHz high speed @ 1.8V pullup"
io8_100m_ft_hs_pd_1v8  "IO8_FT 100MHz high speed @ 1.8V pulldown"
io8_100m_ft_fs_1v8  "IO8_FT 100MHz fast speed @ 1.8V"
io8_100m_ft_fs_pu_1v8  "IO8_FT 100MHz fast speed @ 1.8V pullup"
io8_100m_ft_fs_pd_1v8  "IO8_FT 100MHz fast speed @ 1.8V pulldown"
io8_100m_ft_ms_1v8  "IO8_FT 100MHz med speed @ 1.8V"
io8_100m_ft_ms_pu_1v8  "IO8_FT 100MHz med speed @ 1.8V pullup"
io8_100m_ft_ms_pd_1v8  "IO8_FT 100MHz med speed @ 1.8V pulldown"
io8_100m_ft_ls_1v8  "IO8_FT 100MHz low speed @ 1.8V"
io8_100m_ft_ls_pu_1v8  "IO8_FT 100MHz low speed @ 1.8V pullup"
io8_100m_ft_ls_pd_1v8  "IO8_FT 100MHz low speed @ 1.8V pulldown"
io8_100m_ft_hs_3v3  "IO8_FT 100MHz high speed @ 3.3V"
io8_100m_ft_hs_pu_3v3  "IO8_FT 100MHz high speed @ 3.3V pullup"
io8_100m_ft_hs_pd_3v3  "IO8_FT 100MHz high speed @ 3.3V pulldown"
io8_100m_ft_fs_3v3  "IO8_FT 100MHz fast speed @ 3.3V"
io8_100m_ft_fs_pu_3v3  "IO8_FT 100MHz fast speed @ 3.3V pullup"
io8_100m_ft_fs_pd_3v3  "IO8_FT 100MHz fast speed @ 3.3V pulldown"
io8_100m_ft_ms_3v3  "IO8_FT 100MHz med speed @ 3.3V"
io8_100m_ft_ms_pu_3v3  "IO8_FT 100MHz med speed @ 3.3V pullup"
io8_100m_ft_ms_pd_3v3  "IO8_FT 100MHz med speed @ 3.3V pulldown"
io8_100m_ft_ls_3v3  "IO8_FT 100MHz low speed @ 3.3V"
io8_100m_ft_ls_pu_3v3  "IO8_FT 100MHz low speed @ 3.3V pullup"
io8_100m_ft_ls_pd_3v3  "IO8_FT 100MHz low speed @ 3.3V pulldown"
io8usb_adp "IOUSB ADP @ 3.3V"
io8usb_vbus "IOUSB VBUS @ 3.3V"
[Model Selector] io8_166m_hslv_ft
io8_166m_ft_hs_1v2  "IO8_FT 166MHz high speed @ 1.2V"
io8_166m_ft_hs_pu_1v2  "IO8_FT 166MHz high speed @ 1.2V pullup"
io8_166m_ft_hs_pd_1v2  "IO8_FT 166MHz high speed @ 1.2V pulldown"
io8_166m_ft_fs_1v2  "IO8_FT 166MHz fast speed @ 1.2V"
io8_166m_ft_fs_pu_1v2  "IO8_FT 166MHz fast speed @ 1.2V pullup"
io8_166m_ft_fs_pd_1v2  "IO8_FT 166MHz fast speed @ 1.2V pulldown"
io8_166m_ft_ms_1v2  "IO8_FT 166MHz med speed @ 1.2V"
io8_166m_ft_ms_pu_1v2  "IO8_FT 166MHz med speed @ 1.2V pullup"
io8_166m_ft_ms_pd_1v2  "IO8_FT 166MHz med speed @ 1.2V pulldown"
io8_166m_ft_ls_1v2  "IO8_FT 166MHz low speed @ 1.2V"
io8_166m_ft_ls_pu_1v2  "IO8_FT 166MHz low speed @ 1.2V pullup"
io8_166m_ft_ls_pd_1v2  "IO8_FT 166MHz low speed @ 1.2V pulldown"
io8_166m_ft_hs_1v8  "IO8_FT 166MHz high speed @ 1.8V"
io8_166m_ft_hs_pu_1v8  "IO8_FT 166MHz high speed @ 1.8V pullup"
io8_166m_ft_hs_pd_1v8  "IO8_FT 166MHz high speed @ 1.8V pulldown"
io8_166m_ft_fs_1v8  "IO8_FT 166MHz fast speed @ 1.8V"
io8_166m_ft_fs_pu_1v8  "IO8_FT 166MHz fast speed @ 1.8V pullup"
io8_166m_ft_fs_pd_1v8  "IO8_FT 166MHz fast speed @ 1.8V pulldown"
io8_166m_ft_ms_1v8  "IO8_FT 166MHz med speed @ 1.8V"
io8_166m_ft_ms_pu_1v8  "IO8_FT 166MHz med speed @ 1.8V pullup"
io8_166m_ft_ms_pd_1v8  "IO8_FT 166MHz med speed @ 1.8V pulldown"
io8_166m_ft_ls_1v8  "IO8_FT 166MHz low speed @ 1.8V"
io8_166m_ft_ls_pu_1v8  "IO8_FT 166MHz low speed @ 1.8V pullup"
io8_166m_ft_ls_pd_1v8  "IO8_FT 166MHz low speed @ 1.8V pulldown"
io8_166m_ft_hs_3v3  "IO8_FT 166MHz high speed @ 3.3V"
io8_166m_ft_hs_pu_3v3  "IO8_FT 166MHz high speed @ 3.3V pullup"
io8_166m_ft_hs_pd_3v3  "IO8_FT 166MHz high speed @ 3.3V pulldown"
io8_166m_ft_fs_3v3  "IO8_FT 166MHz fast speed @ 3.3V"
io8_166m_ft_fs_pu_3v3  "IO8_FT 166MHz fast speed @ 3.3V pullup"
io8_166m_ft_fs_pd_3v3  "IO8_FT 166MHz fast speed @ 3.3V pulldown"
io8_166m_ft_ms_3v3  "IO8_FT 166MHz med speed @ 3.3V"
io8_166m_ft_ms_pu_3v3  "IO8_FT 166MHz med speed @ 3.3V pullup"
io8_166m_ft_ms_pd_3v3  "IO8_FT 166MHz med speed @ 3.3V pulldown"
io8_166m_ft_ls_3v3  "IO8_FT 166MHz low speed @ 3.3V"
io8_166m_ft_ls_pu_3v3  "IO8_FT 166MHz low speed @ 3.3V pullup"
io8_166m_ft_ls_pd_3v3  "IO8_FT 166MHz low speed @ 3.3V pulldown"
io8_166m_hslv_ft_hs_1v2  "IO8_FT 166MHz HSLV high speed @ 1.2V"
io8_166m_hslv_ft_hs_pu_1v2  "IO8_FT 166MHz HSLV high speed @ 1.2V pullup"
io8_166m_hslv_ft_hs_pd_1v2  "IO8_FT 166MHz HSLV high speed @ 1.2V pulldown"
io8_166m_hslv_ft_fs_1v2  "IO8_FT 166MHz HSLV fast speed @ 1.2V"
io8_166m_hslv_ft_fs_pu_1v2  "IO8_FT 166MHz HSLV fast speed @ 1.2V pullup"
io8_166m_hslv_ft_fs_pd_1v2  "IO8_FT 166MHz HSLV fast speed @ 1.2V pulldown"
io8_166m_hslv_ft_ms_1v2  "IO8_FT 166MHz HSLV med speed @ 1.2V"
io8_166m_hslv_ft_ms_pu_1v2  "IO8_FT 166MHz HSLV med speed @ 1.2V pullup"
io8_166m_hslv_ft_ms_pd_1v2  "IO8_FT 166MHz HSLV med speed @ 1.2V pulldown"
io8_166m_hslv_ft_ls_1v2  "IO8_FT 166MHz HSLV low speed @ 1.2V"
io8_166m_hslv_ft_ls_pu_1v2  "IO8_FT 166MHz HSLV low speed @ 1.2V pullup"
io8_166m_hslv_ft_ls_pd_1v2  "IO8_FT 166MHz HSLV low speed @ 1.2V pulldown"
io8_166m_hslv_ft_hs_1v8  "IO8_FT 166MHz HSLV high speed @ 1.8V"
io8_166m_hslv_ft_hs_pu_1v8  "IO8_FT 166MHz HSLV high speed @ 1.8V pullup"
io8_166m_hslv_ft_hs_pd_1v8  "IO8_FT 166MHz HSLV high speed @ 1.8V pulldown"
io8_166m_hslv_ft_fs_1v8  "IO8_FT 166MHz HSLV fast speed @ 1.8V"
io8_166m_hslv_ft_fs_pu_1v8  "IO8_FT 166MHz HSLV fast speed @ 1.8V pullup"
io8_166m_hslv_ft_fs_pd_1v8  "IO8_FT 166MHz HSLV fast speed @ 1.8V pulldown"
io8_166m_hslv_ft_ms_1v8  "IO8_FT 166MHz HSLV med speed @ 1.8V"
io8_166m_hslv_ft_ms_pu_1v8  "IO8_FT 166MHz HSLV med speed @ 1.8V pullup"
io8_166m_hslv_ft_ms_pd_1v8  "IO8_FT 166MHz HSLV med speed @ 1.8V pulldown"
io8_166m_hslv_ft_ls_1v8  "IO8_FT 166MHz HSLV low speed @ 1.8V"
io8_166m_hslv_ft_ls_pu_1v8  "IO8_FT 166MHz HSLV low speed @ 1.8V pullup"
io8_166m_hslv_ft_ls_pd_1v8  "IO8_FT 166MHz HSLV low speed @ 1.8V pulldown"
io8_166m_hslv_ft_hs_2v5  "IO8_FT 166MHz HSLV high speed @ 2.5V"
io8_166m_hslv_ft_hs_pu_2v5  "IO8_FT 166MHz HSLV high speed @ 2.5V pullup"
io8_166m_hslv_ft_hs_pd_2v5  "IO8_FT 166MHz HSLV high speed @ 2.5V pulldown"
io8_166m_hslv_ft_fs_2v5  "IO8_FT 166MHz HSLV fast speed @ 2.5V"
io8_166m_hslv_ft_fs_pu_2v5  "IO8_FT 166MHz HSLV fast speed @ 2.5V pullup"
io8_166m_hslv_ft_fs_pd_2v5  "IO8_FT 166MHz HSLV fast speed @ 2.5V pulldown"
io8_166m_hslv_ft_ms_2v5  "IO8_FT 166MHz HSLV med speed @ 2.5V"
io8_166m_hslv_ft_ms_pu_2v5  "IO8_FT 166MHz HSLV med speed @ 2.5V pullup"
io8_166m_hslv_ft_ms_pd_2v5  "IO8_FT 166MHz HSLV med speed @ 2.5V pulldown"
io8_166m_hslv_ft_ls_2v5  "IO8_FT 166MHz HSLV low speed @ 2.5V"
io8_166m_hslv_ft_ls_pu_2v5  "IO8_FT 166MHz HSLV low speed @ 2.5V pullup"
io8_166m_hslv_ft_ls_pd_2v5  "IO8_FT 166MHz HSLV low speed @ 2.5V pulldown"
[Model Selector] io8_spi_hslv_ft
io8_spi_ft_hs_1v2  "IO8_FT SPI high speed @ 1.2V"
io8_spi_ft_hs_pu_1v2  "IO8_FT SPI high speed @ 1.2V pullup"
io8_spi_ft_hs_pd_1v2  "IO8_FT SPI high speed @ 1.2V pulldown"
io8_spi_ft_fs_1v2  "IO8_FT SPI fast speed @ 1.2V"
io8_spi_ft_fs_pu_1v2  "IO8_FT SPI fast speed @ 1.2V pullup"
io8_spi_ft_fs_pd_1v2  "IO8_FT SPI fast speed @ 1.2V pulldown"
io8_spi_ft_ms_1v2  "IO8_FT SPI med speed @ 1.2V"
io8_spi_ft_ms_pu_1v2  "IO8_FT SPI med speed @ 1.2V pullup"
io8_spi_ft_ms_pd_1v2  "IO8_FT SPI med speed @ 1.2V pulldown"
io8_spi_ft_ls_1v2  "IO8_FT SPI low speed @ 1.2V"
io8_spi_ft_ls_pu_1v2  "IO8_FT SPI low speed @ 1.2V pullup"
io8_spi_ft_ls_pd_1v2  "IO8_FT SPI low speed @ 1.2V pulldown"
io8_spi_ft_hs_1v8  "IO8_FT SPI high speed @ 1.8V"
io8_spi_ft_hs_pu_1v8  "IO8_FT SPI high speed @ 1.8V pullup"
io8_spi_ft_hs_pd_1v8  "IO8_FT SPI high speed @ 1.8V pulldown"
io8_spi_ft_fs_1v8  "IO8_FT SPI fast speed @ 1.8V"
io8_spi_ft_fs_pu_1v8  "IO8_FT SPI fast speed @ 1.8V pullup"
io8_spi_ft_fs_pd_1v8  "IO8_FT SPI fast speed @ 1.8V pulldown"
io8_spi_ft_ms_1v8  "IO8_FT SPI med speed @ 1.8V"
io8_spi_ft_ms_pu_1v8  "IO8_FT SPI med speed @ 1.8V pullup"
io8_spi_ft_ms_pd_1v8  "IO8_FT SPI med speed @ 1.8V pulldown"
io8_spi_ft_ls_1v8  "IO8_FT SPI low speed @ 1.8V"
io8_spi_ft_ls_pu_1v8  "IO8_FT SPI low speed @ 1.8V pullup"
io8_spi_ft_ls_pd_1v8  "IO8_FT SPI low speed @ 1.8V pulldown"
io8_spi_ft_hs_3v3  "IO8_FT SPI high speed @ 3.3V"
io8_spi_ft_hs_pu_3v3  "IO8_FT SPI high speed @ 3.3V pullup"
io8_spi_ft_hs_pd_3v3  "IO8_FT SPI high speed @ 3.3V pulldown"
io8_spi_ft_fs_3v3  "IO8_FT SPI fast speed @ 3.3V"
io8_spi_ft_fs_pu_3v3  "IO8_FT SPI fast speed @ 3.3V pullup"
io8_spi_ft_fs_pd_3v3  "IO8_FT SPI fast speed @ 3.3V pulldown"
io8_spi_ft_ms_3v3  "IO8_FT SPI med speed @ 3.3V"
io8_spi_ft_ms_pu_3v3  "IO8_FT SPI med speed @ 1.8V pullup"
io8_spi_ft_ms_pd_3v3  "IO8_FT SPI med speed @ 3.3V pulldown"
io8_spi_ft_ls_3v3  "IO8_FT SPI low speed @ 3.3V"
io8_spi_ft_ls_pu_3v3  "IO8_FT SPI low speed @ 3.3V pullup"
io8_spi_ft_ls_pd_3v3  "IO8_FT SPI low speed @ 3.3V pulldown"
io8_spi_hslv_ft_hs_1v2  "IO8_FT SPI HSLV high speed @ 1.2V"
io8_spi_hslv_ft_hs_pu_1v2  "IO8_FT SPI HSLV high speed @ 1.2V pullup"
io8_spi_hslv_ft_hs_pd_1v2  "IO8_FT SPI HSLV high speed @ 1.2V pulldown"
io8_spi_hslv_ft_fs_1v2  "IO8_FT SPI HSLV fast speed @ 1.2V"
io8_spi_hslv_ft_fs_pu_1v2  "IO8_FT SPI HSLV fast speed @ 1.2V pullup"
io8_spi_hslv_ft_fs_pd_1v2  "IO8_FT SPI HSLV fast speed @ 1.2V pulldown"
io8_spi_hslv_ft_ms_1v2  "IO8_FT SPI HSLV med speed @ 1.2V"
io8_spi_hslv_ft_ms_pu_1v2  "IO8_FT SPI HSLV med speed @ 1.2V pullup"
io8_spi_hslv_ft_ms_pd_1v2  "IO8_FT SPI HSLV med speed @ 1.2V pulldown"
io8_spi_hslv_ft_ls_1v2  "IO8_FT SPI HSLV low speed @ 1.2V"
io8_spi_hslv_ft_ls_pu_1v2  "IO8_FT SPI HSLV low speed @ 1.2V pullup"
io8_spi_hslv_ft_ls_pd_1v2  "IO8_FT SPI HSLV low speed @ 1.2V pulldown"
io8_spi_hslv_ft_hs_1v8  "IO8_FT SPI HSLV high speed @ 1.8V"
io8_spi_hslv_ft_hs_pu_1v8  "IO8_FT SPI HSLV high speed @ 1.8V pullup"
io8_spi_hslv_ft_hs_pd_1v8  "IO8_FT SPI HSLV high speed @ 1.8V pulldown"
io8_spi_hslv_ft_fs_1v8  "IO8_FT SPI HSLV fast speed @ 1.8V"
io8_spi_hslv_ft_fs_pu_1v8  "IO8_FT SPI HSLV fast speed @ 1.8V pullup"
io8_spi_hslv_ft_fs_pd_1v8  "IO8_FT SPI HSLV fast speed @ 1.8V pulldown"
io8_spi_hslv_ft_ms_1v8  "IO8_FT SPI HSLV med speed @ 1.8V"
io8_spi_hslv_ft_ms_pu_1v8  "IO8_FT SPI HSLV med speed @ 1.8V pullup"
io8_spi_hslv_ft_ms_pd_1v8  "IO8_FT SPI HSLV med speed @ 1.8V pulldown"
io8_spi_hslv_ft_ls_1v8  "IO8_FT SPI HSLV low speed @ 1.8V"
io8_spi_hslv_ft_ls_pu_1v8  "IO8_FT SPI HSLV low speed @ 1.8V pullup"
io8_spi_hslv_ft_ls_pd_1v8  "IO8_FT SPI HSLV low speed @ 1.8V pulldown"
io8_spi_hslv_ft_hs_2v5  "IO8_FT SPI HSLV high speed @ 2.5V"
io8_spi_hslv_ft_hs_pu_2v5  "IO8_FT SPI HSLV high speed @ 2.5V pullup"
io8_spi_hslv_ft_hs_pd_2v5  "IO8_FT SPI HSLV high speed @ 2.5V pulldown"
io8_spi_hslv_ft_fs_2v5  "IO8_FT SPI HSLV fast speed @ 2.5V"
io8_spi_hslv_ft_fs_pu_2v5  "IO8_FT SPI HSLV fast speed @ 2.5V pullup"
io8_spi_hslv_ft_fs_pd_2v5  "IO8_FT SPI HSLV fast speed @ 2.5V pulldown"
io8_spi_hslv_ft_ms_2v5  "IO8_FT SPI HSLV med speed @ 2.5V"
io8_spi_hslv_ft_ms_pu_2v5  "IO8_FT SPI HSLV med speed @ 2.5V pullup"
io8_spi_hslv_ft_ms_pd_2v5  "IO8_FT SPI HSLV med speed @ 2.5V pulldown"
io8_spi_hslv_ft_ls_2v5  "IO8_FT SPI HSLV low speed @ 2.5V"
io8_spi_hslv_ft_ls_pu_2v5  "IO8_FT SPI HSLV low speed @ 2.5V pullup"
io8_spi_hslv_ft_ls_pd_2v5  "IO8_FT SPI HSLV low speed @ 2.5V pulldown"
[Model Selector] io8_spi_ft
io8_spi_ft_hs_1v2  "IO8_FT SPI high speed @ 1.2V"
io8_spi_ft_hs_pu_1v2  "IO8_FT SPI high speed @ 1.2V pullup"
io8_spi_ft_hs_pd_1v2  "IO8_FT SPI high speed @ 1.2V pulldown"
io8_spi_ft_fs_1v2  "IO8_FT SPI fast speed @ 1.2V"
io8_spi_ft_fs_pu_1v2  "IO8_FT SPI fast speed @ 1.2V pullup"
io8_spi_ft_fs_pd_1v2  "IO8_FT SPI fast speed @ 1.2V pulldown"
io8_spi_ft_ms_1v2  "IO8_FT SPI med speed @ 1.2V"
io8_spi_ft_ms_pu_1v2  "IO8_FT SPI med speed @ 1.2V pullup"
io8_spi_ft_ms_pd_1v2  "IO8_FT SPI med speed @ 1.2V pulldown"
io8_spi_ft_ls_1v2  "IO8_FT SPI low speed @ 1.2V"
io8_spi_ft_ls_pu_1v2  "IO8_FT SPI low speed @ 1.2V pullup"
io8_spi_ft_ls_pd_1v2  "IO8_FT SPI low speed @ 1.2V pulldown"
io8_spi_ft_hs_1v8  "IO8_FT SPI high speed @ 1.8V"
io8_spi_ft_hs_pu_1v8  "IO8_FT SPI high speed @ 1.8V pullup"
io8_spi_ft_hs_pd_1v8  "IO8_FT SPI high speed @ 1.8V pulldown"
io8_spi_ft_fs_1v8  "IO8_FT SPI fast speed @ 1.8V"
io8_spi_ft_fs_pu_1v8  "IO8_FT SPI fast speed @ 1.8V pullup"
io8_spi_ft_fs_pd_1v8  "IO8_FT SPI fast speed @ 1.8V pulldown"
io8_spi_ft_ms_1v8  "IO8_FT SPI med speed @ 1.8V"
io8_spi_ft_ms_pu_1v8  "IO8_FT SPI med speed @ 1.8V pullup"
io8_spi_ft_ms_pd_1v8  "IO8_FT SPI med speed @ 1.8V pulldown"
io8_spi_ft_ls_1v8  "IO8_FT SPI low speed @ 1.8V"
io8_spi_ft_ls_pu_1v8  "IO8_FT SPI low speed @ 1.8V pullup"
io8_spi_ft_ls_pd_1v8  "IO8_FT SPI low speed @ 1.8V pulldown"
io8_spi_ft_hs_3v3  "IO8_FT SPI high speed @ 3.3V"
io8_spi_ft_hs_pu_3v3  "IO8_FT SPI high speed @ 3.3V pullup"
io8_spi_ft_hs_pd_3v3  "IO8_FT SPI high speed @ 3.3V pulldown"
io8_spi_ft_fs_3v3  "IO8_FT SPI fast speed @ 3.3V"
io8_spi_ft_fs_pu_3v3  "IO8_FT SPI fast speed @ 3.3V pullup"
io8_spi_ft_fs_pd_3v3  "IO8_FT SPI fast speed @ 3.3V pulldown"
io8_spi_ft_ms_3v3  "IO8_FT SPI med speed @ 3.3V"
io8_spi_ft_ms_pu_3v3  "IO8_FT SPI med speed @ 1.8V pullup"
io8_spi_ft_ms_pd_3v3  "IO8_FT SPI med speed @ 3.3V pulldown"
io8_spi_ft_ls_3v3  "IO8_FT SPI low speed @ 3.3V"
io8_spi_ft_ls_pu_3v3  "IO8_FT SPI low speed @ 3.3V pullup"
io8_spi_ft_ls_pd_3v3  "IO8_FT SPI low speed @ 3.3V pulldown"
io8_spi_hslv_ft_hs_1v2  "IO8_FT SPI HSLV high speed @ 1.2V"
io8_spi_hslv_ft_hs_pu_1v2  "IO8_FT SPI HSLV high speed @ 1.2V pullup"
io8_spi_hslv_ft_hs_pd_1v2  "IO8_FT SPI HSLV high speed @ 1.2V pulldown"
io8_spi_hslv_ft_fs_1v2  "IO8_FT SPI HSLV fast speed @ 1.2V"
io8_spi_hslv_ft_fs_pu_1v2  "IO8_FT SPI HSLV fast speed @ 1.2V pullup"
io8_spi_hslv_ft_fs_pd_1v2  "IO8_FT SPI HSLV fast speed @ 1.2V pulldown"
io8_spi_hslv_ft_ms_1v2  "IO8_FT SPI HSLV med speed @ 1.2V"
io8_spi_hslv_ft_ms_pu_1v2  "IO8_FT SPI HSLV med speed @ 1.2V pullup"
io8_spi_hslv_ft_ms_pd_1v2  "IO8_FT SPI HSLV med speed @ 1.2V pulldown"
io8_spi_hslv_ft_ls_1v2  "IO8_FT SPI HSLV low speed @ 1.2V"
io8_spi_hslv_ft_ls_pu_1v2  "IO8_FT SPI HSLV low speed @ 1.2V pullup"
io8_spi_hslv_ft_ls_pd_1v2  "IO8_FT SPI HSLV low speed @ 1.2V pulldown"
io8_spi_hslv_ft_hs_1v8  "IO8_FT SPI HSLV high speed @ 1.8V"
io8_spi_hslv_ft_hs_pu_1v8  "IO8_FT SPI HSLV high speed @ 1.8V pullup"
io8_spi_hslv_ft_hs_pd_1v8  "IO8_FT SPI HSLV high speed @ 1.8V pulldown"
io8_spi_hslv_ft_fs_1v8  "IO8_FT SPI HSLV fast speed @ 1.8V"
io8_spi_hslv_ft_fs_pu_1v8  "IO8_FT SPI HSLV fast speed @ 1.8V pullup"
io8_spi_hslv_ft_fs_pd_1v8  "IO8_FT SPI HSLV fast speed @ 1.8V pulldown"
io8_spi_hslv_ft_ms_1v8  "IO8_FT SPI HSLV med speed @ 1.8V"
io8_spi_hslv_ft_ms_pu_1v8  "IO8_FT SPI HSLV med speed @ 1.8V pullup"
io8_spi_hslv_ft_ms_pd_1v8  "IO8_FT SPI HSLV med speed @ 1.8V pulldown"
io8_spi_hslv_ft_ls_1v8  "IO8_FT SPI HSLV low speed @ 1.8V"
io8_spi_hslv_ft_ls_pu_1v8  "IO8_FT SPI HSLV low speed @ 1.8V pullup"
io8_spi_hslv_ft_ls_pd_1v8  "IO8_FT SPI HSLV low speed @ 1.8V pulldown"
io8_spi_hslv_ft_hs_2v5  "IO8_FT SPI HSLV high speed @ 2.5V"
io8_spi_hslv_ft_hs_pu_2v5  "IO8_FT SPI HSLV high speed @ 2.5V pullup"
io8_spi_hslv_ft_hs_pd_2v5  "IO8_FT SPI HSLV high speed @ 2.5V pulldown"
io8_spi_hslv_ft_fs_2v5  "IO8_FT SPI HSLV fast speed @ 2.5V"
io8_spi_hslv_ft_fs_pu_2v5  "IO8_FT SPI HSLV fast speed @ 2.5V pullup"
io8_spi_hslv_ft_fs_pd_2v5  "IO8_FT SPI HSLV fast speed @ 2.5V pulldown"
io8_spi_hslv_ft_ms_2v5  "IO8_FT SPI HSLV med speed @ 2.5V"
io8_spi_hslv_ft_ms_pu_2v5  "IO8_FT SPI HSLV med speed @ 2.5V pullup"
io8_spi_hslv_ft_ms_pd_2v5  "IO8_FT SPI HSLV med speed @ 2.5V pulldown"
io8_spi_hslv_ft_ls_2v5  "IO8_FT SPI HSLV low speed @ 2.5V"
io8_spi_hslv_ft_ls_pu_2v5  "IO8_FT SPI HSLV low speed @ 2.5V pullup"
io8_spi_hslv_ft_ls_pd_2v5  "IO8_FT SPI HSLV low speed @ 2.5V pulldown"
[Define Package Model]  481-tfbga-7x7-ldo-169-220908
[Manufacturer]  unknown
[OEM]  unknown
[Description]  unknown
[Number Of Pins]  150
[Pin Numbers]
| Pin Name Terminal   Net Name   Starting Node   Ending Node
H3 | NRST
M1 | OPAMP1_VINM
H5 | OPAMP2_VINM
K3 | PA0
L3 | PA1
M2 | PA2
N2 | PA3
N1 | PA4
K4 | PA5
N4 | PA6
J5 | PA7
G7 | PA8
G11 | PA9
F11 | PA10
G13 | PA11
F13 | PA12
F12 | PA13
C10 | PA14
A10 | PA15
K5 | PB0
N5 | PB1
L5 | PB2
D6 | PB3
B6 | PB4
C6 | PB5
B5 | PB6
F5 | PB7
E5 | PB8
D5 | PB9
K9 | PB10
L9 | PB11
L10 | PB12
N13 | PB13
M12 | PB14
L11 | PB15
J2 | PC0
J3 | PC1
J4 | PC2
K1 | PC3
L4 | PC4
M4 | PC5
H13 | PC6
G12 | PC7
G10 | PC8
G9 | PC9
C9 | PC10
A9 | PC11
E8 | PC12
E3 | PC13
D1 | PC14-OSC32_IN
E1 | PC15-OSC32_OUT
B9 | PD0
F6 | PD1
F7 | PD2
D8 | PD3
C8 | PD4
E7 | PD5
B7 | PD6
D7 | PD7
L12 | PD8
L13 | PD9
K11 | PD10
M13 | PD11
K10 | PD12
K12 | PD13
J10 | PD14
J11 | PD15
D4 | PE0
C4 | PE1
A1 | PE2
D3 | PE3
C2 | PE4
D2 | PE5
E4 | PE6
L7 | PE7
K7 | PE8
J7 | PE9
H8 | PE10
M8 | PE11
N8 | PE12
L8 | PE13
K8 | PE14
M9 | PE15
E2 | PF0
F3 | PF1
F4 | PF2
G5 | PF3
G6 | PF4
G4 | PF5
H6 | PF6
G2 | PF7
F1 | PF8
G3 | PF9
H4 | PF10
M5 | PF11
K6 | PF12
M6 | PF13
L6 | PF14
N6 | PF15
J6 | PG0
H7 | PG1
K13 | PG2
J8 | PG3
H11 | PG4
J9 | PG5
H10 | PG6
G8 | PG7
H9 | PG8
A7 | PG9
C7 | PG10
M10 | PG11
E6 | PG12
N10 | PG13
N9 | PG14
A5 | PG15
H1 | PH0-OSC_IN
J1 | PH1-OSC_OUT
F10 | PH2
C5 | PH3-BOOT0
E10 | PH4
F9 | PH5
E11 | PH6
F8 | PH7
D12 | PH8
E9 | PH9
C13 | PH10
D9 | PH11
B13 | PH12
C12 | PH13
C11 | PH14
A13 | PH15
B12 | PI0
A12 | PI1
D11 | PI2
D10 | PI3
B10 | PI4
B3 | PI5
A2 | PI6
C3 | PI7
N11 | VCAP
A4 | VCAP
C1 | VBAT
A3 | VDD
L2 | VDDA
H12 | VDDIO2
A6 | VDDIO2
E13 | VDDUSB
L1 | VREFP
B2 | VSS
K2 | VSSA
|[Merged Pins]  A3
|A8  |  VDD
|A11  |  VDD
|B1  |  VDD
|D13  |  VDD
|G1  |  VDD
|J13  |  VDD
|N3  |  VDD
|N7  |  VDD
|N12  |  VDD
|[Merged Pins]  B2
|B4  |  VSS
|B8  |  VSS
|B11  |  VSS
|E12  |  VSS
|F2  |  VSS
|H2  |  VSS
|J12  |  VSS
|M3  |  VSS
|M7  |  VSS
|M11  |  VSS
[Model Data]
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[End Model Data]
[End Package Model]
| Models and submodels in the file (265): io8_100m_ft_hs_1v2 (I/O), io8_100m_ft_hs_pu_1v2 (I/O), io8_100m_ft_hs_pd_1v2 (I/O), io8_100m_ft_fs_1v2 (I/O), io8_100m_ft_fs_pu_1v2 (I/O), io8_100m_ft_fs_pd_1v2 (I/O), io8_100m_ft_ms_1v2 (I/O), io8_100m_ft_ms_pu_1v2 (I/O), io8_100m_ft_ms_pd_1v2 (I/O), io8_100m_ft_ls_1v2 (I/O), io8_100m_ft_ls_pu_1v2 (I/O), io8_100m_ft_ls_pd_1v2 (I/O), io8_100m_ft_hs_1v8 (I/O), io8_100m_ft_hs_pu_1v8 (I/O), io8_100m_ft_hs_pd_1v8 (I/O), io8_100m_ft_fs_1v8 (I/O), io8_100m_ft_fs_pu_1v8 (I/O), io8_100m_ft_fs_pd_1v8 (I/O), io8_100m_ft_ms_1v8 (I/O), io8_100m_ft_ms_pu_1v8 (I/O), io8_100m_ft_ms_pd_1v8 (I/O), io8_100m_ft_ls_1v8 (I/O), io8_100m_ft_ls_pu_1v8 (I/O), io8_100m_ft_ls_pd_1v8 (I/O), io8_100m_ft_hs_3v3 (I/O), io8_100m_ft_hs_pu_3v3 (I/O), io8_100m_ft_hs_pd_3v3 (I/O), io8_100m_ft_fs_3v3 (I/O), io8_100m_ft_fs_pu_3v3 (I/O), io8_100m_ft_fs_pd_3v3 (I/O), io8_100m_ft_ms_3v3 (I/O), io8_100m_ft_ms_pu_3v3 (I/O), io8_100m_ft_ms_pd_3v3 (I/O), io8_100m_ft_ls_3v3 (I/O), io8_100m_ft_ls_pu_3v3 (I/O), io8_100m_ft_ls_pd_3v3 (I/O), io8_100m_hslv_ft_hs_1v2 (I/O), io8_100m_hslv_ft_hs_pu_1v2 (I/O), io8_100m_hslv_ft_hs_pd_1v2 (I/O), io8_100m_hslv_ft_fs_1v2 (I/O), io8_100m_hslv_ft_fs_pu_1v2 (I/O), io8_100m_hslv_ft_fs_pd_1v2 (I/O), io8_100m_hslv_ft_ms_1v2 (I/O), io8_100m_hslv_ft_ms_pu_1v2 (I/O), io8_100m_hslv_ft_ms_pd_1v2 (I/O), io8_100m_hslv_ft_ls_1v2 (I/O), io8_100m_hslv_ft_ls_pu_1v2 (I/O), io8_100m_hslv_ft_ls_pd_1v2 (I/O), io8_100m_hslv_ft_hs_1v8 (I/O), io8_100m_hslv_ft_hs_pu_1v8 (I/O), io8_100m_hslv_ft_hs_pd_1v8 (I/O), io8_100m_hslv_ft_fs_1v8 (I/O), io8_100m_hslv_ft_fs_pu_1v8 (I/O), io8_100m_hslv_ft_fs_pd_1v8 (I/O), io8_100m_hslv_ft_ms_1v8 (I/O), io8_100m_hslv_ft_ms_pu_1v8 (I/O), io8_100m_hslv_ft_ms_pd_1v8 (I/O), io8_100m_hslv_ft_ls_1v8 (I/O), io8_100m_hslv_ft_ls_pu_1v8 (I/O), io8_100m_hslv_ft_ls_pd_1v8 (I/O), io8_100m_hslv_ft_hs_2v5 (I/O), io8_100m_hslv_ft_hs_pu_2v5 (I/O), io8_100m_hslv_ft_hs_pd_2v5 (I/O), io8_100m_hslv_ft_fs_2v5 (I/O), io8_100m_hslv_ft_fs_pu_2v5 (I/O), io8_100m_hslv_ft_fs_pd_2v5 (I/O), io8_100m_hslv_ft_ms_2v5 (I/O), io8_100m_hslv_ft_ms_pu_2v5 (I/O), io8_100m_hslv_ft_ms_pd_2v5 (I/O), io8_100m_hslv_ft_ls_2v5 (I/O), io8_100m_hslv_ft_ls_pu_2v5 (I/O), io8_100m_hslv_ft_ls_pd_2v5 (I/O), io8_100m_i2c_ft_1v2 (I/O_open_drain), io8_100m_i2c_ft_pu_1v2 (I/O_open_drain), io8_100m_i2c_ft_pd_1v2 (I/O_open_drain), io8_100m_i2c_ft_1v8 (I/O_open_drain), io8_100m_i2c_ft_pu_1v8 (I/O_open_drain), io8_100m_i2c_ft_pd_1v8 (I/O_open_drain), io8_100m_i2c_ft_3v3 (I/O_open_drain), io8_100m_i2c_ft_pu_3v3 (I/O_open_drain)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
